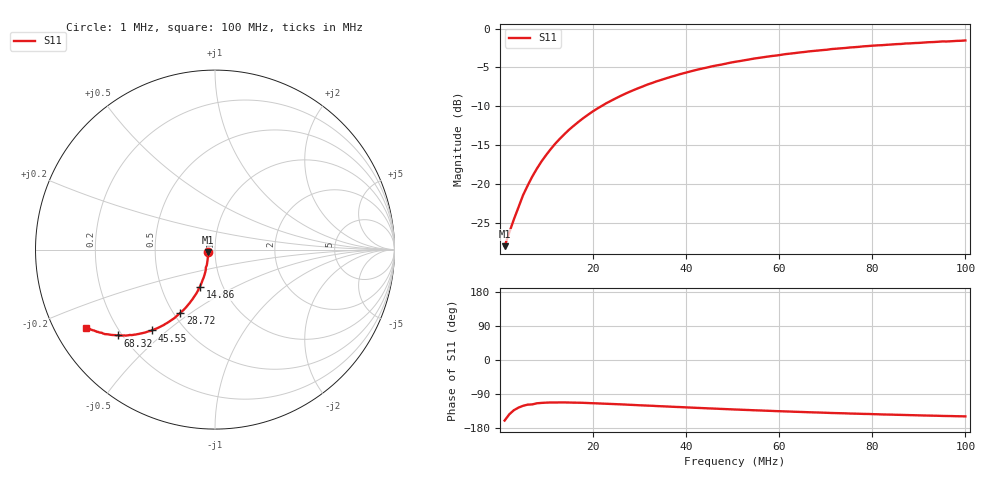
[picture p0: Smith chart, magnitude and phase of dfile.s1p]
# Hz S RI R 50.0
! written by SimSmith version 18.3b
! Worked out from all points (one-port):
!   101 points, 1 MHz to 100 MHz, reference 50 ohm
!   lowest |S11| = -28.0 dB at 1 MHz (marker M1), VSWR 1.08, Z = 46.4 - j1.28 ohm
!   |S11| at or under -10 dB: start of sweep to 21.75 MHz
!   S11 on the Smith chart (normalised r, x): 1 MHz: 0.93, -0.03; 14.86 MHz: 0.78, -0.34; 28.72 MHz: 0.54, -0.46; 45.55 MHz: 0.33, -0.44; 68.32 MHz: 0.18, -0.37; 100 MHz: 0.09, -0.28
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1000000  -0.0373 -0.0137
2980000  -0.0399 -0.0435
4960000  -0.0435 -0.0726
6940000  -0.0509 -0.0992
8920000  -0.055 -0.1282
9910000  -0.0588 -0.1417
1.189e7  -0.0686 -0.1684
1.387e7  -0.0783 -0.1943
1.486e7  -0.0846 -0.207
1.783e7  -0.1032 -0.2433
1.981e7  -0.1186 -0.266
2.278e7  -0.1416 -0.2981
2.575e7  -0.1661 -0.3268
2.872e7  -0.1927 -0.3528
3.367e7  -0.2393 -0.3904
3.862e7  -0.2857 -0.4203
4.555e7  -0.352 -0.4502
5.05e7  -0.3979 -0.4639
5.743e7  -0.4577 -0.4754
6.337e7  -0.5055 -0.4781
6.832e7  -0.5416 -0.478
7.525e7  -0.5899 -0.4731
7.921e7  -0.6124 -0.4712
8.218e7  -0.6308 -0.4632
8.812e7  -0.662 -0.4551
9.505e7  -0.6978 -0.4434
9.604e7  -0.6991 -0.4402
1e8  -0.7173 -0.435
